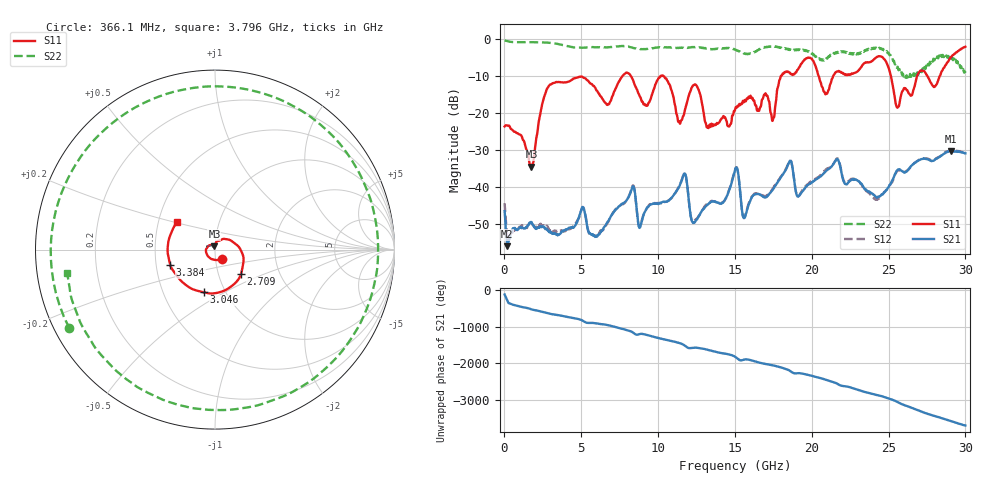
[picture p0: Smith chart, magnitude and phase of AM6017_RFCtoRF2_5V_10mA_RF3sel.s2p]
!Agilent Technologies,E8364B,MY43040894,A.07.50.67
!Agilent E8364B: A.07.50.67
!Date: Tuesday, August 21, 2018 13:38:07
!Correction: S11(Full 2 Port(1,2))
!S21(Full 2 Port(1,2))
!S12(Full 2 Port(1,2))
!S22(Full 2 Port(1,2))
!S2P File: Measurements: S11, S21, S12, S22:
# Hz S  dB  R 50
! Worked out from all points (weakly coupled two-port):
!   1601 points, 10 MHz to 30 GHz, reference 50 ohm
!   highest |S21| = -30.23 dB at 29.08 GHz (marker M1); lowest = -55.9 dB at 178.7 MHz (marker M2)
!   lowest |S11| = -34.5 dB at 1.753 GHz (marker M3), VSWR 1.04, Z = 49.7 + j1.85 ohm
!   |S11| at or under -10 dB: start of sweep to 7.676 GHz; 8.233 GHz to 10.15 GHz (1.918 GHz wide, 20.9 % of centre); 10.35 GHz to 17.99 GHz (7.635 GHz wide, 53.9 % of centre)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
!   |S22| runs from -10.4 to -0.3 dB; largest |S21 - S12| = 0.0074
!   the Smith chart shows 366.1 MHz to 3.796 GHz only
!   S11 on the Smith chart (normalised r, x): 366.1 MHz: 1.07, -0.11; 2.709 GHz: 1.28, -0.36; 3.046 GHz: 0.79, -0.40; 3.384 GHz: 0.59, -0.11; 3.796 GHz: 0.63, +0.21
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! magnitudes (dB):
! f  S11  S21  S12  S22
! 10 MHz  -23.6  -46.4  -44.3  -0.3
! 178.7 MHz  -23.3  -55.9  -53.0  -0.5
! 366.1 MHz  -23.9  -53.8  -53.0  -0.7
! 1.753 GHz  -34.5  -49.4  -49.6  -0.8
! 2.709 GHz  -14.0  -51.3  -50.7  -0.9
! 3.046 GHz  -12.2  -52.2  -51.7  -1.0
! 3.384 GHz  -11.6  -52.7  -51.8  -1.3
! 3.796 GHz  -11.7  -51.8  -52.0  -1.6
! 5.015 GHz  -10.1  -45.9  -46.0  -2.3
! 10.02 GHz  -10.6  -44.5  -44.3  -2.2
! 11.41 GHz  -22.7  -39.6  -39.4  -2.3
! 12.34 GHz  -12.4  -49.6  -49.1  -2.1
! 13.28 GHz  -24.0  -44.5  -44.2  -2.6
! 15.01 GHz  -19.1  -35.3  -35.2  -2.9
! 15.62 GHz  -16.6  -48.3  -48.0  -3.9
! 17.46 GHz  -21.9  -40.7  -40.4  -2.0
! 20.01 GHz  -5.3  -38.8  -38.3  -3.8
! 20.91 GHz  -14.8  -35.7  -35.2  -5.6
! 25.01 GHz  -7.9  -39.8  -39.7  -3.8
! 25.6 GHz  -18.5  -35.3  -35.5  -7.5
! 29.08 GHz  -4.8  -30.2  -30.1  -5.3
! 30 GHz  -2.0  -30.9  -30.9  -9.1
